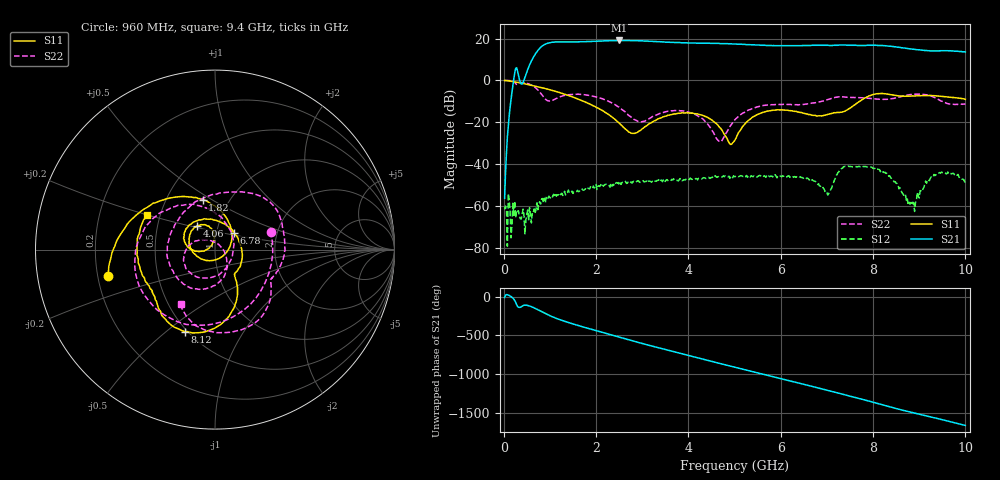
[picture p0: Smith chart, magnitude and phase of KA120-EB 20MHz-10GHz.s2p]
!Agilent	"Technologies,N5230A,MY45001650,A.07.50.48"
!Agilent	N5230A:	A.07.50.48
!Date:	"Wednesday,"	August	"04,"	2021	8:24:08
!Correction:	S11(Full	2	"Port(1,2))"
!S21(Full	2	"Port(1,2))"
!S12(Full	2	"Port(1,2))"
!S22(Full	2	"Port(1,2))"
!S2P	File:	Measurements:	"S11,"	"S21,"	"S12,"	S22:
#	Hz	S	dB	R	50
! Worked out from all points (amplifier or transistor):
!   500 points, 20 MHz to 10 GHz, reference 50 ohm
!   highest |S21| = 19.1 dB at 2.5 GHz (marker M1)
!   |S21| within 3 dB of that: 815 MHz to 8.46 GHz (7.645 GHz wide, 165 % of centre)
!   unconditionally stable (mu >= 1): start of sweep to 95.41 MHz; 102.2 MHz to end of sweep
!   at 1.68 GHz: K = 17.61, MAG = 20.1 dB, |S12| = -52.6 dB
!   at 5.02 GHz: K = 13.12, MAG = 17.5 dB, |S12| = -45.9 dB
!   at 10 GHz: K = 25.72, MAG = 14.5 dB, |S12| = -49.7 dB
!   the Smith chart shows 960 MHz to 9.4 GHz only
!   S11 on the Smith chart (normalised r, x): 960 MHz: 0.24, -0.12; 1.82 GHz: 0.75, +0.45; 4.06 GHz: 0.79, +0.22; 6.78 GHz: 1.21, +0.23; 8.12 GHz: 0.49, -0.58; 9.4 GHz: 0.42, +0.20
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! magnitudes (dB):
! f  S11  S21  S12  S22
! 20 MHz  0.0  -56.3  -61.6  0.0
! 120 MHz  -0.3  -16.8  -56.9  -0.1
! 240 MHz  -0.7  3.7  -57.7  -0.9
! 400 MHz  -1.3  -1.7  -63.8  -1.0
! 960 MHz  -4.2  17.8  -56.3  -9.8
! 1.7 GHz  -9.7  18.5  -51.9  -6.7
! 1.82 GHz  -10.9  18.6  -51.5  -7.1
! 2.5 GHz  -20.4  19.1  -50.0  -12.8
! 3.36 GHz  -18.2  18.5  -47.5  -16.0
! 4.06 GHz  -15.6  17.9  -47.1  -15.6
! 4.68 GHz  -22.5  17.6  -46.0  -29.1
! 5.02 GHz  -28.1  17.4  -45.9  -18.5
! 5.62 GHz  -15.2  16.8  -46.1  -12.0
! 6.68 GHz  -16.6  16.8  -47.5  -10.8
! 6.78 GHz  -17.0  16.8  -49.0  -10.5
! 7.02 GHz  -16.2  16.8  -54.8  -9.2
! 7.38 GHz  -14.8  16.9  -41.2  -7.9
! 8.12 GHz  -6.3  16.7  -42.5  -9.0
! 8.34 GHz  -6.6  16.4  -45.8  -8.9
! 8.88 GHz  -7.5  14.9  -58.5  -6.6
! 9.4 GHz  -7.4  14.1  -44.6  -9.0
! 10 GHz  -9.0  13.6  -49.7  -11.2
